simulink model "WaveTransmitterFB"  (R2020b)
settings: Solver=FixedStepDiscrete  StartTime=0.0  StopTime=inf  RelTol=1e-3
PreLoadFcn:
  | platform = sdruExampleFindRadio;
  | sdrqpsktx = sdruqpsktransmitter_init(platform, false);
  | clear platform
PostLoadFcn:
  | sdruExampleSetAvailableRadio;
InitFcn:
  | platform = get_param([gcs '/USRP Transmitter'], 'Platform');
  | sdrqpsktx = sdruqpsktransmitter_init(platform, false);
  | clear platform
libraries: sdrublksprivate x1, dspsrcs4 x1, commsdrhw_v2 x1

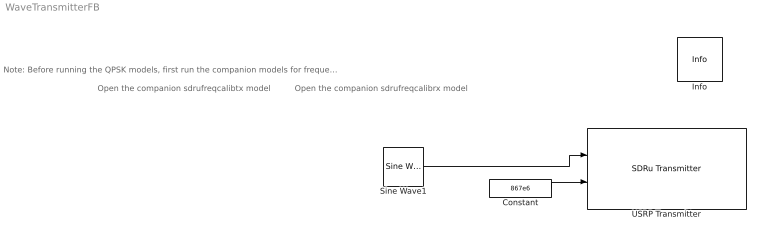
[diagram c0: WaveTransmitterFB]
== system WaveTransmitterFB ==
  note: Note: Before running the QPSK models, first run the companion models for frequency offset calibration.
  note: Open the companion sdrufreqcalibrx model
  note: Open the companion sdrufreqcalibtx model
  Constant : Constant  Value=867e6
  Info : sdrublksprivate/Info  SystemSampleTime=-1  VariantActivationTime=update diagram  Latency=0  AutoFrameSizeCalculation=off
  Sine Wave1 : dspsrcs4/Sine Wave  Amplitude=1  Frequency=100  Phase=0  SampleMode=Discrete  OutComplex=Complex  CompMethod=Trigonometric fcn  TableSize=Speed  SampleTime=1/1000  SamplesPerFrame=1  ResetState=Restart at time zero  OutputFrames=off  dataType=double  wordLen=16  udDataType=sfix(16)  fracBitsMode=Best precision  numFracBits=15  OutDataTypeStr=double  LastOutDataTypeStr=double
  USRP Transmitter : commsdrhw_v2/SDRu Transmitter  rxtx=tx  initializeIPAddress=0  devMap=0  USRP2_IP=192.168.10.3  USRP_IP_X300=192.168.10.2  USRP_IP_X310=192.168.30.2  USRP_IP_N300=No devices found  USRP_IP_N310=192.168.10.2  USRP_IP_N320=No devices found  USRP_serialNumB200=30B2ACA  USRP_serialNumB210=ECR04ZDBT  platform=N200/N210/USRP2  prevPlatform=N200/N210/USRP2  lastIPAddressPopup=192.168.10.2  USRP_ID=192.168.10.3  LastIPAddress=192.168.10.2  ChannelMapping=1  centerFrequencySrc=Input port  centerFrequency=867e6  loOffsetSrc=Dialog  loOffset=0  gainSrc=Dialog  gain=30  PPSSource=Internal  clockSource=Internal  masterClkRateParam=100e6  masterClkRateB200=sdrqpsktx.MasterClockRate  masterClkRateB210=sdrqpsktx.MasterClockRate  masterClkRateX300=200e6  masterClkRateX310=200e6  masterClkRateN300=125e6  masterClkRateN310=125e6  masterClkRateN320=200e6  decimInterpSrc=Dialog  lastDecimSource=Dialog  decimInterp=sdrqpsktx.USRPInterpolationFactor  USRP2_IP_NUM=[49 57 50 46 49 54 56 46 49 48 46 51]  frameLength=362  sampleRate=2000000  TransportDataType=int16  outputDatatype=Same as transport data type  overrunUnderrunPort=off  sampleTime=1  dboardInfo=|  HOST_DATA_PORT=30000  HOST_CONTROL_PORT=30001  USRP2_DATA_PORT=32769  USRP2_CONTROL_PORT=32768  bufferMode=Continuous streaming  EnableBurstMode=off  NumFramesInBurst=100
      | dbid: 0
      |           dbName: 'no db found'
      |          freqMin: 0
      |          freqMax: 0
      |          gainMin: 0
      |          gainMax: 0
      |     gainStepSize: 0
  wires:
  Sine Wave1/1 -> USRP Transmitter/1
  Constant/1 -> USRP Transmitter/2
